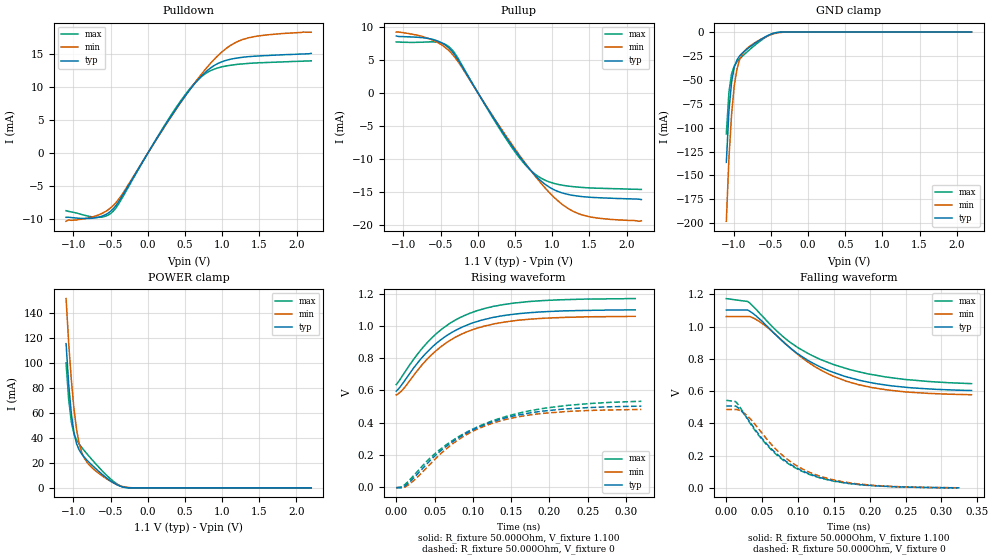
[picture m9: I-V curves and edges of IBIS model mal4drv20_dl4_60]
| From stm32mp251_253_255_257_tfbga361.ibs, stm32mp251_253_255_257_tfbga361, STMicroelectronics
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[Model] mal4drv20_dl4_60
Model_type   I/O
Polarity   Non-Inverting
Enable   Active-High
C_comp   1.837pF   1.837pF   1.849pF
C_comp_pullup   942.491fF   934.703fF   950.576fF
C_comp_pulldown 782.742fF   781.933fF   799.826fF
Vinh = 310.000mV
Vinl = 190.000mV
Vmeas = 250.000mV
Vref = 0.00V
Rref = 50Ohms
Cref = 0pF
[Model Spec]
Vinh   310.000mV   301.000mV   326.000mV
Vinl   190.000mV   181.000mV   206.000mV
Vmeas   250.000mV   241.000mV   266.000mV
Vref   0.00V   0.00V   0.00V
D_overshoot_ampl_h 0.3 NA   NA
D_overshoot_ampl_l 0.3 NA   NA
D_overshoot_area_l 100.000m NA   NA
D_overshoot_area_h 100.000m NA   NA
[Receiver Thresholds]
Vth = 250.000mV
Vth_min = 241.000mV
Vth_max = 266.000mV
Vinh_ac = 600.000mV
Vinh_dc = 600.000mV
Vinl_ac = -600.000mV
Vinl_dc = -600.000mV
Tslew_ac = 5.000ns
Threshold_sensitivity = 0.5
Reference_supply Pullup_ref
[Temperature Range]   25.000   125.000   -40.000
[Voltage Range]   1.100V   1.060V   1.170V
[GND Clamp Reference]   0.00V   0.00V   0.00V
[C Comp Corner]
| variable   typ   min   max
C_comp 1.849pF   1.837pF   1.837pF
C_comp_pullup 942.491fF   950.576fF   934.703fF
C_comp_pulldown 781.933fF   799.826fF   782.742fF
[Pulldown Reference]   0.00V   0.00V   0.00V
[POWER Clamp Reference]   1.100V   1.060V   1.170V
[Pullup Reference]   1.100V   1.060V   1.170V
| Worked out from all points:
|   slope of the pulldown table from 0 to 0.165 V, typ, clamps not added: 54.9 ohm
|   slope of the pullup table from 0 to 0.165 V, typ, clamps not added: 54.9 ohm
|   GND clamp passes 1 mA (typ) near -0.45 V on its own axis
|   POWER clamp passes 1 mA (typ) near -0.36 V on its own axis
|   rising waveform, R_fixture 50.000Ohm, V_fixture 1.100: 20-80 % time 72.9ps typ, 72.4ps min, 72.9ps max; typ from 0.596 V to 1.1 V
|   rising waveform, R_fixture 50.000Ohm, V_fixture 0: 20-80 % time 92.4ps typ, 84.4ps min, 105ps max; typ from -0.002 V to 0.503 V
|   falling waveform, R_fixture 50.000Ohm, V_fixture 1.100: 20-80 % time 101ps typ, 94.7ps min, 109ps max; typ from 1.1 V to 0.604 V
|   falling waveform, R_fixture 50.000Ohm, V_fixture 0: 20-80 % time 74.6ps typ, 74.6ps min, 74.2ps max; typ from 0.508 V to 0.001 V
[GND Clamp]
-1.099V   -136.3mA   -197.9mA   -106.5mA
-1.064V   -82.47mA   -132mA     -62.93mA
-1.028V   -52.05mA   -85.75mA   -43.61mA
-992.7mV  -36.88mA   -56.43mA   -35.5mA
-957.3mV  -29.36mA   -39.14mA   -31.26mA
-921.8mV  -25.1mA    -29.22mA   -28.2mA
-886.4mV  -22.16mA   -23.33mA   -25.51mA
-850.9mV  -19.73mA   -19.54mA   -22.95mA
-780mV    -15.43mA   -14.59mA   -18.04mA
-531.8mV  -3.288mA   -3.748mA   -3.604mA
-390mV    -251.1uA   -613.4uA   -163.8uA
2.198V    42.3nA     621.2nA    4.643nA
[Power Clamp]
-1.098V   115.5mA    151.6mA    100.1mA
-1.063V   83.06mA    116mA      70.82mA
-1.027V   59.24mA    86.19mA    52.7mA
-991.8mV  44.02mA    63.02mA    43.29mA
-956.4mV  35.26mA    46.38mA    38.3mA
-920.9mV  30.19mA    35.27mA    34.98mA
-885.5mV  26.87mA    28.15mA    32.19mA
-850mV    24.29mA    23.52mA    29.6mA
-672.7mV  13.97mA    12.28mA    17.45mA
-424.5mV  2.786mA    2.91mA     3.554mA
-282.7mV  160.9uA    380.1uA    143.1uA
2.199V    -14.13nA   -533.6nA   -2.884nA
[Pulldown]
-1.099V   -9.7mA     -10.3mA    -8.7mA
-673.6mV  -9.711mA   -9.385mA   -9.71mA
-567.3mV  -9.288mA   -8.812mA   -9.526mA
-460.9mV  -8.363mA   -7.872mA   -8.732mA
-319.1mV  -6.023mA   -5.784mA   -6.273mA
106.4mV   1.95mA     1.9mA      2.021mA
425.4mV   7.453mA    7.379mA    7.643mA
673.6mV   11.08mA    11.27mA    11.1mA
886.4mV   13.22mA    14.12mA    12.69mA
1.099V    14.18mA    16.21mA    13.28mA
1.312V    14.56mA    17.32mA    13.55mA
2.198V    15.1mA     18.3mA     13.97mA
[Pullup]
-1.098V   8.6mA      9.2mA      7.699mA
-601.8mV  8.07mA     7.95mA     7.709mA
-460mV    7.402mA    7.047mA    7.429mA
-353.6mV  6.363mA    5.969mA    6.608mA
426.4mV   -7.516mA   -7.319mA   -7.781mA
639.1mV   -10.81mA   -10.7mA    -10.94mA
816.4mV   -13.04mA   -13.27mA   -12.72mA
958.2mV   -14.29mA   -15.09mA   -13.51mA
1.1V      -15.06mA   -16.61mA   -13.94mA
1.348V    -15.68mA   -18.3mA    -14.31mA
1.632V    -15.92mA   -19.03mA   -14.48mA
2.199V    -16.2mA    -19.41mA   -14.66mA
[Ramp]
R_load=50.000Ohm
dV/dt_r   302.910mV/84.500ps  291.688mV/80.000ps  322.320mV/92.000ps
dV/dt_f   302.910mV/90.000ps  291.688mV/87.000ps  322.320mV/95.500ps
[Rising waveform]
R_fixture=50.000Ohm
V_fixture=1.100
V_fixture_min=1.060
V_fixture_max=1.170
0s        596mV      572.2mV    636.4mV
11ps      660.9mV    618.7mV    711.7mV
28ps      771.6mV    725.8mV    826.2mV
49ps      877.9mV    833.9mV    937.3mV
72ps      958mV      915.5mV    1.022V
101ps     1.02V      978.7mV    1.087V
136ps     1.061V     1.019V     1.129V
173ps     1.081V     1.041V     1.151V
218ps     1.093V     1.052V     1.162V
312ps     1.099V     1.059V     1.169V
[Rising waveform]
R_fixture=50.000Ohm
V_fixture=0
0s        -2.469mV   -1.391mV   -2.908mV
8ps       -2.469mV   -1.391mV   4.356mV
17ps      30.62mV    19.01mV    43.32mV
45ps      170.2mV    148mV      185.1mV
70ps      270.6mV    256.5mV    279.5mV
98ps      351.2mV    342.5mV    356.7mV
129ps     411.4mV    402.2mV    417.7mV
167ps     455.2mV    443.4mV    467.1mV
214ps     483.2mV    467.4mV    502.9mV
320ps     502.9mV    482.6mV    532.8mV
[Falling waveform]
R_fixture=50.000Ohm
V_fixture=1.100
V_fixture_min=1.060
V_fixture_max=1.170
0s        1.102V     1.062V     1.173V
30ps      1.102V     1.062V     1.155V
39ps      1.075V     1.05V      1.118V
55ps      1.01V      1.003V     1.042V
88ps      871mV      871.6mV    905.3mV
119ps     777.3mV    764.2mV    821.6mV
149ps     716.6mV    692.7mV    765.4mV
183ps     669.6mV    641.5mV    721.9mV
223ps     637.5mV    608mV      687.4mV
342ps     603.7mV    577.7mV    646.4mV
[Falling waveform]
R_fixture=50.000Ohm
V_fixture=0
0s        507.8mV    486.2mV    543.3mV
13ps      507.8mV    486.2mV    535mV
27ps      445.4mV    456.3mV    444mV
49ps      311.3mV    343.3mV    304.6mV
69ps      216.4mV    240.9mV    210.1mV
89ps      147.3mV    164.7mV    142.6mV
115ps     88.51mV    99.51mV    85.21mV
143ps     50.45mV    56.79mV    49.22mV
178ps     25.16mV    28.13mV    24.34mV
325ps     1.221mV    1.494mV    1.192mV
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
